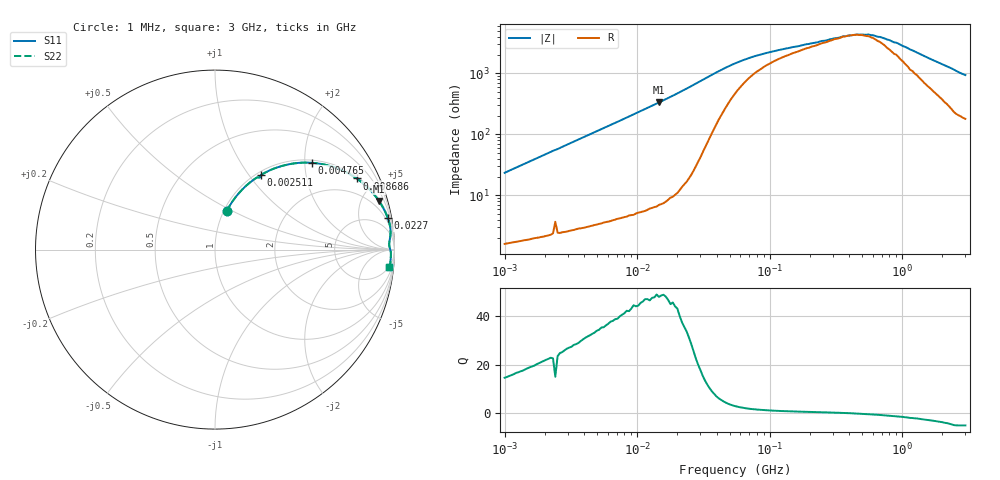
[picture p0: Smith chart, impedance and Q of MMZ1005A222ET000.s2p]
! S-parameter Generated by TDK Corporation
! Copyright(C) 2016 TDK Corporation.
! All Rights Reserved.
! TDK P/N: MMZ1005A222ET000 (Chip Beads)
! Property: |Z|=2200¶ at 100MHz
! Size(LxWxT): 1x0.5x0.5mm, 0.039x0.02x0.02inches
! Model Type: s2p (Touchstone File Format Version 1.0)
! Frequency: DC=Yes Start=1MHz Stop=3000MHz 202points Log-sweep
! Note: This model was converted from impedance.
! Model Generated on May. 16, 2016
! Hash(MD5):
! Port Assignments:
!  1 ---@@@--- 2
! Applicable Conditions:
!  Temperature = 25 degC
!  DC Bias Current = 0 A
!  Small Signal Operation
! Terms and conditions regarding TDK Simulation Models
! (1)This simulation model is being provided solely for informational purposes. Please refer to the specifications of the products in terms of detailed characteristics of such products.
! (2)In no event shall TDK Corporation of any of its subsidiaries be liable for any loss or damage arising, directly or indirectly,
!  From any information contained in this simulation model, including, but not limited to loss or damages arising from any inaccuracies, omissions or errors in connection with such information.
! (3)Any and all copyrights on this simulation model are owned by TDK Corporation.
!  Duplication or redistribution of this simulation model without prior written permission from TDK Corporation is prohibited.
! (4)This simulation model is subject to any modification or change without any prior notice.
! (5)Neither TDK Corporation nor any of its subsidiaries shall make any warranty, express or implied,
!  Including but not limited to the correctness, implied warranties of merchantability and fitness for a particular purpose with respect to this simulation models.
! (6)The use of this simulation model shall be deemed to have consented to the terms and conditions hereof.
# MHz S MA R 50
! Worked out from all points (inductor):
!   201 points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, 1 MHz to 3 GHz, reference 50 ohm
!   read as one part in series: L = 3.72 uH near 1.041 MHz
!   highest Q = 48.5 at 14.62 MHz (marker M1), where L = 3.64 uH
!   self-resonance near 416.3 MHz
!   S11 on the Smith chart (normalised r, x): 1 MHz: 1.03, +0.47; 2.511 MHz: 1.05, +1.15; 4.765 MHz: 1.07, +2.17; 8.686 MHz: 1.09, +3.93; 22.7 MHz: 1, +11; 3 GHz: 5, -18
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1  0.2249 73.1  0.9592 -13.0  0.9592 -13.0  0.2249 73.1
1.616692  0.3466 66.8  0.9202 -20.3  0.9202 -20.3  0.3466 66.8
2.511129  0.49 58.3  0.8511 -29.3  0.8511 -29.3  0.49 58.3
3.900413  0.6546 47.3  0.7348 -40.9  0.7348 -40.9  0.6546 47.3
4.764734  0.7241 41.9  0.6682 -46.4  0.6682 -46.4  0.7241 41.9
6.305767  0.8094 34.5  0.5661 -54.0  0.5661 -54.0  0.8094 34.5
8.686058  0.883 26.7  0.4489 -62.0  0.4489 -62.0  0.883 26.7
11.04425  0.9219 21.6  0.3679 -67.2  0.3679 -67.2  0.9219 21.6
14.61624  0.9526 16.6  0.285 -72.2  0.285 -72.2  0.9526 16.6
22.70269  0.9783 10.5  0.1815 -77.9  0.1815 -77.9  0.9783 10.5
35.26298  0.9837 6.2  0.1082 -78.3  0.1082 -78.3  0.9837 6.2
54.77226  0.9767 3.6  0.0668 -67.8  0.0668 -67.8  0.9767 3.6
72.48696  0.973 2.6  0.0529 -58.0  0.0529 -58.0  0.973 2.6
95.93103  0.9712 2.0  0.04442 -48.7  0.04442 -48.7  0.9712 2.0
213.6344  0.9726 0.8  0.03075 -26.8  0.03075 -26.8  0.9726 0.8
359.4878  0.9763 0.2  0.02399 -8.3  0.02399 -8.3  0.9763 0.2
457.0858  0.9776 -0.1  0.02247 5.5  0.02247 5.5  0.9776 -0.1
558.3748  0.9789 -0.4  0.02244 19.9  0.02244 19.9  0.9789 -0.4
682.1091  0.9795 -0.8  0.02467 33.6  0.02467 33.6  0.9795 -0.8
800.5644  0.9803 -1.1  0.02775 44.3  0.02775 44.3  0.9803 -1.1
1645.649  0.9801 -3.1  0.05692 67.9  0.05692 67.9  0.9801 -3.1
3000  0.975 -5.8  0.1035 73.1  0.1035 73.1  0.975 -5.8
